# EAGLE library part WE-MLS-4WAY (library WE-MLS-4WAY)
Multiline EMI Suppression Ferrite - Filter for common mode or differential mode - High rated current with typ. 4 A - High impedance common mode inductor with 2x2 winding made by PCB line connection - Broardband litering because of the NiZn-ferrite core - RF- common mode inductor for 2,3 or 4 lines in one component -- Perfect suitable for absorption of common or differential mode interferences in the field of EMC -- High current DC output filters of power supplies e.g. battery chargers, industrial power supplies -- With one turn the component performes like a 3 or 4 times common mode chock for the signal
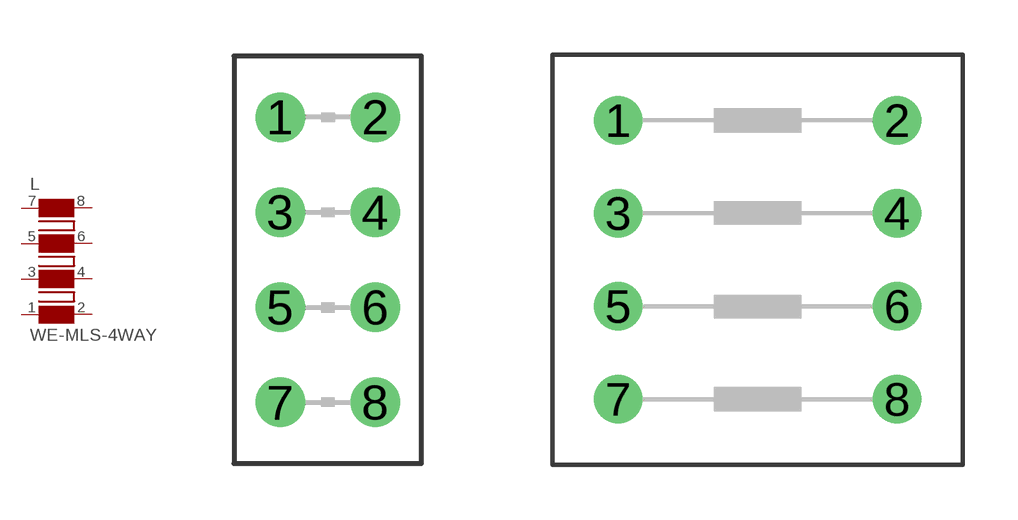
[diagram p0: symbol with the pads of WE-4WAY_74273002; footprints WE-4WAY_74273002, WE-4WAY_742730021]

Designator prefix L

## WE-MLS-4WAY_74273002, WE-MLS-4WAY-74273002_74273002 (MPN: 74273002; OC_FARNELL: 1635787; OC_NEWARK: 08P2349; PACKAGE: 74273002x; SUPPLIER: Wuerth Elektronik)  [WE-4WAY_74273002]
1  4  pas
2  5  pas
3  3  pas
4  6  pas
5  2  pas
6  7  pas
7  1  pas
8  8  pas

## WE-MLS-4WAY_742730021  [WE-4WAY_742730021]
Pads as for WE-4WAY_74273002

## WE-MLS-4WAY_742730022, WE-MLS-4WAY-742730022_742730022 (MPN: 742730022; OC_FARNELL: 1635788; OC_NEWARK: 08P2350; PACKAGE: 74273002x; SUPPLIER: Wuerth Elektronik)  [WE-4WAY_742730022]
Pads as for WE-4WAY_74273002

## WE-MLS-4WAY_742730023  [WE-4WAY_742730023]
Pads as for WE-4WAY_74273002

## Footprint WE-4WAY_74273002 (pad centres in mm)
Multiline EMI Suppression Ferrite WE-MLS
drill 0.813: 1 -1.27,3.81; 2 1.27,3.81; 3 -1.27,1.27; 4 1.27,1.27; 5 -1.27,-1.27; 6 1.27,-1.27; 7 -1.27,-3.81; 8 1.27,-3.81

## Footprint WE-4WAY_742730021 (pad centres in mm)
Multiline EMI Suppression Ferrite WE-MLS
drill 0.813: 1 -3.81,3.81; 2 3.81,3.81; 3 -3.81,1.27; 4 3.81,1.27; 5 -3.81,-1.27; 6 3.81,-1.27; 7 -3.81,-3.81; 8 3.81,-3.81

## Footprint WE-4WAY_742730022 (pad centres in mm)
Multiline EMI Suppression Ferrite WE-MLS
drill 0.813: 1 -3.81,3.81; 2 3.81,3.81; 3 -3.81,1.27; 4 3.81,1.27; 5 -3.81,-1.27; 6 3.81,-1.27; 7 -3.81,-3.81; 8 3.81,-3.81

## Footprint WE-4WAY_742730023 (pad centres in mm)
Multiline EMI Suppression Ferrite WE-MLS
drill 0.813: 1 -3.81,3.81; 2 3.81,3.81; 3 -3.81,1.27; 4 3.81,1.27; 5 -3.81,-1.27; 6 3.81,-1.27; 7 -3.81,-3.81; 8 3.81,-3.81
